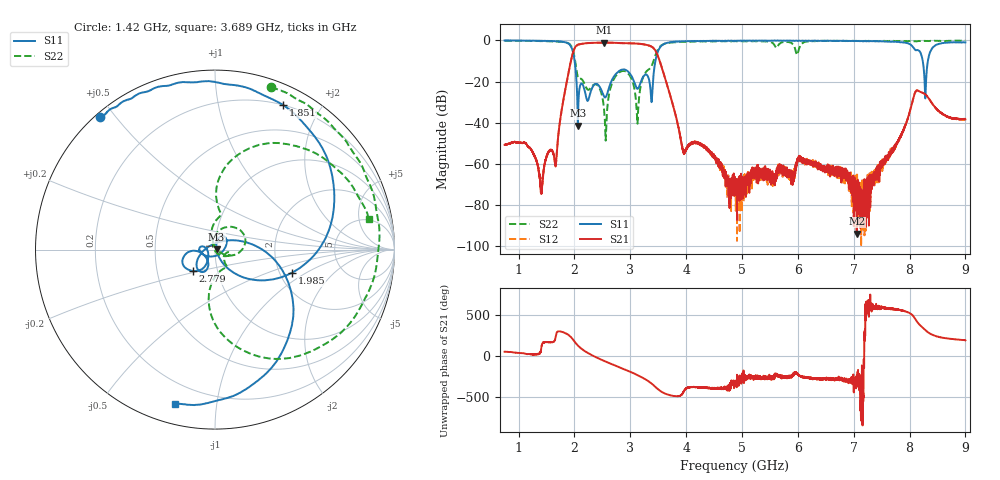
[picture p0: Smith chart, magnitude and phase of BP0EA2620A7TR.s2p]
!Agilent Technologies,E8358A,US41080443,A.07.50.56
!Agilent E8358A: A.07.50.56
!Date: Friday, November 20, 2015 10:49:17
!Correction: S11(Full 2 Port(1,2))
!S21(Full 2 Port(1,2))
!S12(Full 2 Port(1,2))
!S22(Full 2 Port(1,2))
!S2P File: Measurements: S11, S21, S12, S22:
# Hz S  dB  R 50
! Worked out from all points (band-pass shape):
!   6401 points, 750 MHz to 9 GHz, reference 50 ohm
!   highest |S21| = -1.08 dB at 2.529 GHz (marker M1); lowest = -94.0 dB at 7.054 GHz (marker M2)
!   |S21| within 3 dB of the highest: 1.998 GHz to 3.427 GHz (1.429 GHz wide, 52.7 % of centre)
!   lowest |S11| = -41.4 dB at 2.061 GHz (marker M3), VSWR 1.02, Z = 50.9 + j0.0703 ohm
!   |S11| at or under -10 dB: 2.003 GHz to 3.45 GHz (1.447 GHz wide, 53.1 % of centre); 8.237 GHz to 8.328 GHz (91.79 MHz wide, 1.11 % of centre)
!   |S22| runs from -48.7 to -0.1 dB; largest |S21 - S12| = 0.0057
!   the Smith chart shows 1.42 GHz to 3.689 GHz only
!   S11 on the Smith chart (normalised r, x): 1.42 GHz: 0.01, +0.46; 1.851 GHz: 0.20, +1.56; 1.985 GHz: 2.33, -0.75; 2.779 GHz: 0.76, -0.19; 3.689 GHz: 0.10, -0.77
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7.5e8  -0.04 162.3  -50.79 55.6  -50.80 55.6  -0.18 133.2
1.420312e9  -0.19 130.8  -71.28 147.9  -70.85 144.6  -0.34 70.9
1.669102e9  -0.45 105.2  -59.98 -104.0  -59.83 -99.3  -0.52 32.9
1.850859e9  -1.01 64.7  -21.65 -80.6  -21.70 -80.7  -0.99 -13.0
1.984922e9  -6.99 -16.8  -5.00 -164.3  -5.02 -164.2  -5.95 -82.4
2.060977e9  -41.43 4.7  -2.12 131.8  -2.14 131.8  -17.80 -81.0
2.12543e9  -20.95 54.5  -1.65 93.0  -1.68 93.0  -18.77 -54.8
2.313633e9  -23.32 -154.0  -1.21 12.9  -1.25 12.9  -22.33 -10.4
2.528906e9  -27.11 179.8  -1.08 -55.9  -1.12 -55.9  -33.09 -60.3
2.778984e9  -15.32 -136.1  -1.26 -127.1  -1.29 -127.0  -16.11 54.3
3.124453e9  -23.48 -147.6  -1.52 131.2  -1.56 131.3  -39.66 14.5
3.21082e9  -18.72 -112.3  -1.78 100.8  -1.82 100.8  -19.39 100.2
3.500859e9  -5.00 -39.1  -7.96 -46.6  -8.03 -46.5  -4.10 68.2
3.689062e9  -1.04 -104.5  -24.42 -113.5  -24.39 -113.7  -1.18 11.3
3.957188e9  -0.48 -139.8  -54.35 -73.2  -54.32 -68.2  -0.70 -32.5
4.875e9  -0.17 176.7  -73.30 -9.5  -66.64 13.5  -0.37 -107.9
6.25043e9  -0.11 179.4  -59.08 93.3  -59.19 89.8  -0.42 -169.1
7.053516e9  -0.36 164.6  -94.02 53.5  -69.53 109.2  -0.24 166.7
7.625859e9  -0.60 138.7  -56.72 -137.7  -55.67 -133.4  -0.32 153.1
8.13375e9  -4.67 92.7  -24.30 64.7  -24.35 65.0  -0.44 140.5
8.32582e9  -10.44 -158.7  -27.53 -63.5  -27.52 -63.6  -0.27 135.8
9e9  -0.98 96.7  -38.38 -163.6  -38.35 -161.9  -0.15 120.1
